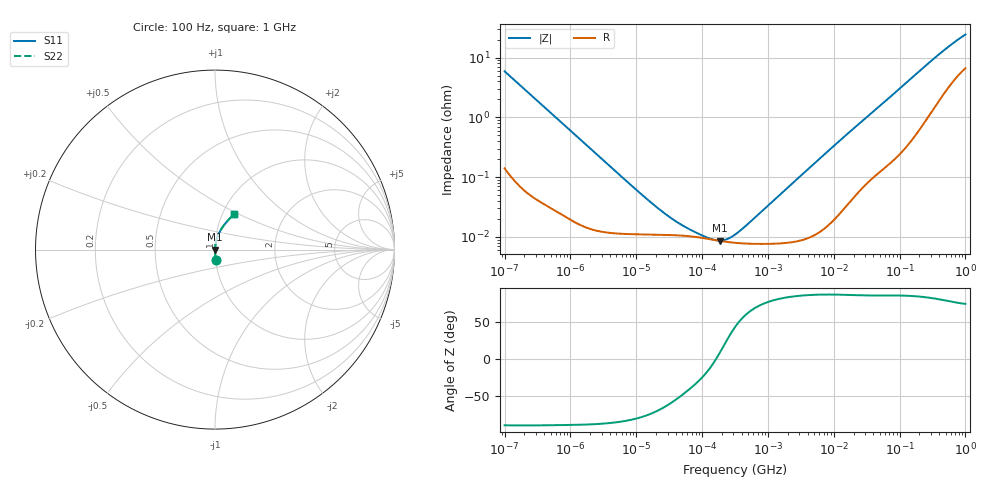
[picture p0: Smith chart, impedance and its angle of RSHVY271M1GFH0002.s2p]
! RSHVY271M1GFH0002  S-PARAMETER MODEL  (General Type)
! Model Generated by ELNA Corporation (https://www.yuden.co.jp/en/)
! Version 1.0
! ELNA Control No. 231222
! Copyright (c) 2023 ELNA CO.,LTD. All Rights Reserved.
! Products Name : CONDUCTIVE POLYMER HYBRID ALUMINUM ELECTROLYTIC CAPACITORS
! Characteristics :
!  Capacitance  :  270uF  ,  Rated voltage  :  35V
!  Operating Temp. Range  :  -55 to +150 degC  ,  Endurance  :  2000hr at 150 degC
!  Dimension D  :  10mm  ,  Dimension L  :  10mm
! Frequency Range : 100Hz - 1GHz
! External Node Assignments :
!  1  o---| |---o  2
# MHz S RI R 50
!Freq[MHz].  S11 Real  S11 Imag  S21 Real  S21 Imag  S12 Real  S12 Imag  S22 Real  S22 Imag
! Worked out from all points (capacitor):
!   401 points, 100 Hz to 1 GHz, reference 50 ohm
!   read as one part in series: C = 270 uF near 108 Hz
!   lowest |Z| = 8.69 mohm at 187.3 kHz (marker M1)
!   series resonance near 162.3 kHz, so ESL is about 3.6 nH
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0.0001  0.00483 -0.0585  0.9952 0.0585  0.9952 0.0585  0.00483 -0.0585
0.000113  0.00387 -0.0519  0.9961 0.0519  0.9961 0.0519  0.00387 -0.0519
0.000309  0.000782 -0.0191  0.9992 0.0191  0.9992 0.0191  0.000782 -0.0191
0.001488  0.00017 -0.00404  0.9998 0.00404  0.9998 0.00404  0.00017 -0.00404
0.009495  0.000111 -0.000635  0.9999 0.000635  0.9999 0.000635  0.000111 -0.000635
0.022131  0.000109 -0.000271  0.9999 0.000271  0.9999 0.000271  0.000109 -0.000271
0.031805  0.000108 -0.000187  0.9999 0.000187  0.9999 0.000187  0.000108 -0.000187
0.043904  0.000106 -0.000134  0.9999 0.000134  0.9999 0.000134  0.000106 -0.000134
0.063096  0.000103 -8.85e-05  0.9999 8.85e-05  0.9999 8.85e-05  0.000103 -8.85e-05
0.094406  9.72e-05 -4.92e-05  0.9999 4.92e-05  0.9999 4.92e-05  9.72e-05 -4.92e-05
0.120226  9.31e-05 -2.75e-05  0.9999 2.75e-05  0.9999 2.75e-05  9.31e-05 -2.75e-05
0.187284  8.57e-05 1.41e-05  0.9999 -1.41e-05  0.9999 -1.41e-05  8.57e-05 1.41e-05
0.269153  8.11e-05 5.4e-05  0.9999 -5.4e-05  0.9999 -5.4e-05  8.11e-05 5.4e-05
0.316228  7.96e-05 7.44e-05  0.9999 -7.44e-05  0.9999 -7.44e-05  7.96e-05 7.44e-05
0.512861  7.7e-05 0.000151  0.9999 -0.000151  0.9999 -0.000151  7.7e-05 0.000151
4.704354  0.000104 0.00157  0.9999 -0.00157  0.9999 -0.00157  0.000104 0.00157
15.75796  0.000359 0.00515  0.9996 -0.00515  0.9996 -0.00515  0.000359 0.00515
69.9842  0.0021 0.0212  0.9979 -0.0212  0.9979 -0.0212  0.0021 0.0212
176.8072  0.00776 0.0516  0.9922 -0.0516  0.9922 -0.0516  0.00776 0.0516
380.1894  0.028 0.1025  0.972 -0.1025  0.972 -0.1025  0.028 0.1025
668.3439  0.0653 0.155  0.9347 -0.155  0.9347 -0.155  0.0653 0.155
1000  0.105 0.1961  0.895 -0.1961  0.895 -0.1961  0.105 0.1961
